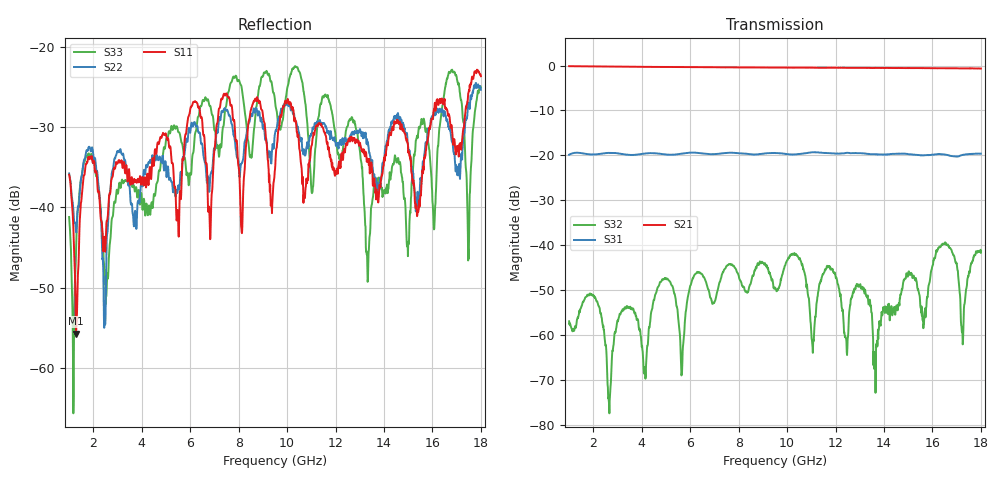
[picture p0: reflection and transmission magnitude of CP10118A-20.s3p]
! Amtery
! Email: info@amtery.com
! Phone: 886-2-2883-7839
! Model Number: CP10118A-20
! 3-port S-parameter measurement data for Directional Coupler
! Frequency Range: 1 GHz to 18 GHz
! Port 1: Input
! Port 2: Output
! Port 3: Coupled
# Hz S db R 50
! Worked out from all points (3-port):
!   1361 points, 1 GHz to 18 GHz, reference 50 ohm
!   strongest paths, dB at 1 GHz, 5.25 GHz, 9.5 GHz, 13.75 GHz, 18 GHz:
!     S21: -0.1, -0.3, -0.5, -0.5, -0.7
!     S31: -19.9, -19.9, -19.5, -19.8, -19.6
!     S32: -56.9, -49.0, -49.4, -58.8, -41.6
!   lowest |S11| = -55.7 dB at 1.288 GHz (marker M1), VSWR 1.00, Z = 49.9 + j0.124 ohm
!   |S11| at or under -10 dB: start of sweep to end of sweep
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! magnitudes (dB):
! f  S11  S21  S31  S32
! 1 GHz  -35.9  -0.1  -19.9  -56.9
! 1.288 GHz  -55.7  -0.2  -19.4  -58.0
! 2.663 GHz  -38.4  -0.2  -19.4  -77.4
! 4.875 GHz  -30.7  -0.3  -19.7  -47.5
! 5.662 GHz  -34.7  -0.3  -19.6  -68.0
! 6.25 GHz  -26.9  -0.4  -19.4  -46.2
! 9.5 GHz  -35.3  -0.5  -19.5  -49.4
! 13.01 GHz  -32.0  -0.5  -19.5  -48.7
! 13.64 GHz  -37.3  -0.5  -19.7  -64.2
! 18 GHz  -23.7  -0.7  -19.6  -41.6
